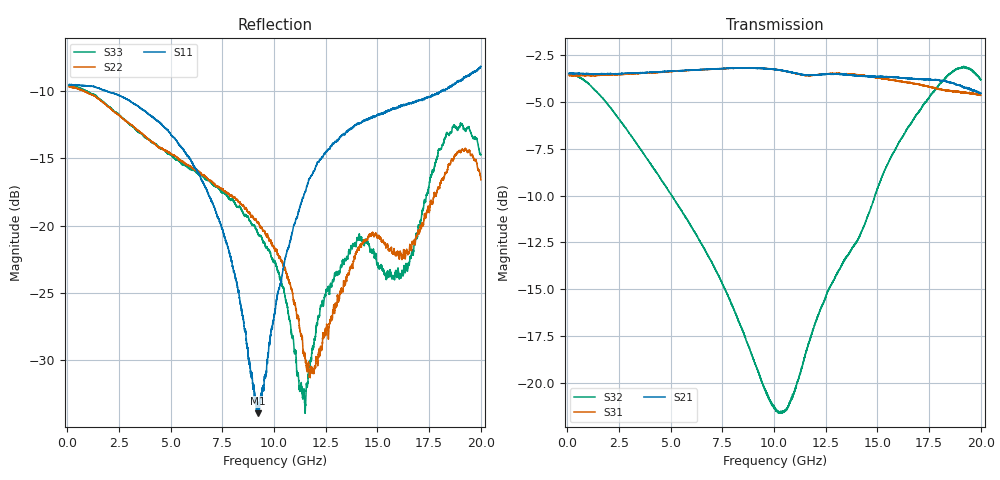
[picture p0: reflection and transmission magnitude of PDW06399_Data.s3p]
# Hz S MA R  50
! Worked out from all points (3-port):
!   6401 points, 100 MHz to 20 GHz, reference 50 ohm
!   strongest paths, dB at 100 MHz, 5.075 GHz, 10.05 GHz, 15.03 GHz, 20 GHz:
!     S21: -3.5, -3.3, -3.2, -3.6, -4.5
!     S31: -3.6, -3.4, -3.2, -3.7, -4.6
!     S32: -3.5, -10.0, -21.4, -9.6, -3.8
!   lowest |S11| = -33.9 dB at 9.207 GHz (marker M1), VSWR 1.04, Z = 51.1 - j1.72 ohm
!   |S11| at or under -10 dB: 1.930812 GHz to 1.932938 GHz (2.125 MHz wide, 0.11 % of centre); 1.935 GHz to 18.08 GHz (16.14 GHz wide, 161 % of centre)
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1e8  0.3346 178.5  0.672 -1.6  0.6625 -1.6
     0.6718 -1.5  0.3283 175.8  0.668 -2.8
     0.6638 -1.6  0.6692 -2.8  0.3321 175.9
2.323203e9  0.3087 142.7  0.6704 -35.3  0.6651 -35.6
            0.6697 -35.3  0.2634 91.4  0.5231 -58.5
            0.6655 -35.7  0.5238 -58.6  0.2651 90.8
6.337406e9  0.1569 71.8  0.6864 -97.6  0.6866 -99.3
            0.6869 -97.6  0.1593 -20.3  0.2438 -131.5
            0.6857 -99.4  0.2435 -131.6  0.1554 -22.7
9.207359e9  0.02009 -56.9  0.6925 -145.3  0.6933 -148.0
            0.6941 -145.3  0.1027 -77.1  0.1084 159.1
            0.6941 -148.1  0.1083 159.1  0.094 -77.7
1.005e10  0.04882 -137.2  0.6886 -159.9  0.6868 -162.9
          0.6886 -159.9  0.08121 -93.1  0.08543 121.4
          0.6887 -163.0  0.08554 121.8  0.07317 -92.2
1.14617e10  0.1308 -178.6  0.6652 176.6  0.6633 173.1
            0.6649 176.5  0.03264 -93.1  0.1157 43.9
            0.6641 173.0  0.1162 44.1  0.02388 -52.6
1.2951e10  0.2057 143.2  0.668 151.9  0.6694 147.8
           0.669 151.8  0.05035 -58.5  0.1912 -12.8
           0.6701 147.8  0.1909 -12.8  0.06628 -42.9
1.50716e10  0.26 104.2  0.6574 114.6  0.6536 108.6
            0.6588 114.5  0.09143 -119.5  0.3387 -54.4
            0.6537 108.5  0.3375 -54.4  0.06996 -127.6
1.73259e10  0.2984 76.1  0.6465 73.1  0.6202 67.0
            0.6461 72.9  0.1076 113.2  0.5621 -111.0
            0.6225 66.8  0.5639 -111.0  0.1224 85.4
2e10  0.391 52.9  0.5958 20.5  0.5871 17.1
      0.5947 20.4  0.1481 -24.2  0.6447 163.0
      0.5875 17.1  0.6464 163.1  0.1834 -30.5
